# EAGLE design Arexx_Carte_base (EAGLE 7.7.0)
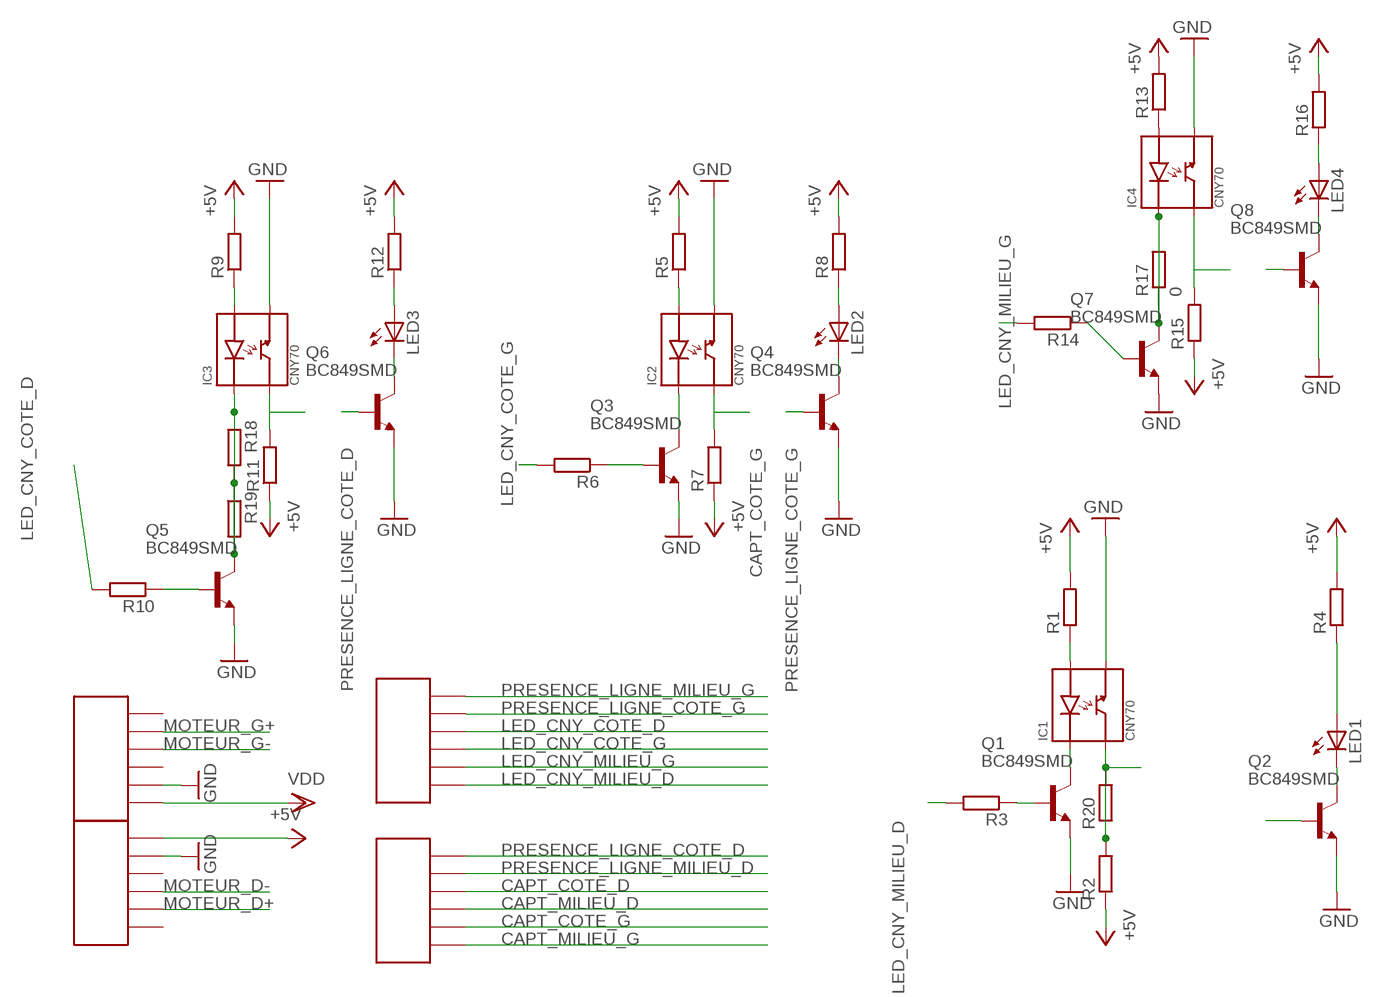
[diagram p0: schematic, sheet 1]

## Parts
IC1  CNY70  [CNY70]
IC2  CNY70  [CNY70]
IC3  CNY70  [CNY70]
IC4  CNY70  [CNY70]
LED1  LED5MM  [LED5MM]
LED2  LED5MM  [LED5MM]
LED3  LED5MM  [LED5MM]
LED4  LED5MM  [LED5MM]
Q1  BC849SMD  [SOT23-BEC]
Q2  BC849SMD  [SOT23-BEC]
Q3  BC849SMD  [SOT23-BEC]
Q4  BC849SMD  [SOT23-BEC]
Q5  BC849SMD  [SOT23-BEC]
Q6  BC849SMD  [SOT23-BEC]
Q7  BC849SMD  [SOT23-BEC]
Q8  BC849SMD  [SOT23-BEC]
R1  R-EU_R1206  [R1206]
R2  R-EU_R1206  [R1206]
R3  R-EU_R1206  [R1206]
R4  R-EU_R1206  [R1206]
R5  R-EU_R1206  [R1206]
R6  R-EU_R1206  [R1206]
R7  R-EU_R1206  [R1206]
R8  R-EU_R1206  [R1206]
R9  R-EU_R1206  [R1206]
R10  R-EU_R1206  [R1206]
R11  R-EU_R1206  [R1206]
R12  R-EU_R1206  [R1206]
R13  R-EU_R1206  [R1206]
R14  R-EU_R1206  [R1206]
R15  R-EU_R1206  [R1206]
R16  R-EU_R1206  [R1206]
R17  0  R-EU_R1206  [R1206]
R18  R-EU_R1206  [R1206]
R19  R-EU_R1206  [R1206]
R20  R-EU_R1206  [R1206]
U$1  AREXX_CONNECTEUR  [AREXX_CONNECTEUR]
U$2  AREXX_CONNECTEUR  [AREXX_CONNECTEUR]
U$3  AREXX_CONNECTEUR  [AREXX_CONNECTEUR]
U$4  AREXX_CONNECTEUR  [AREXX_CONNECTEUR]

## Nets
+5V: R1.2 R2.1 R4.2 R5.2 R7.1 R8.2 R9.2 R11.1 R12.2 R13.2 R15.1 R16.2 U$3.P$1
CAPT_COTE_D: IC3.DC R11.2 U$4.P$3
CAPT_COTE_G: IC2.DC R7.2 U$4.P$5
CAPT_MILIEU_D: IC1.DC R2.2 R20.1 R20.2 U$4.P$4
CAPT_MILIEU_G: IC4.DC R15.2 U$4.P$6
GND: IC1.DE IC2.DE IC3.DE IC4.DE Q1.E Q2.E Q3.E Q4.E Q5.E Q6.E Q7.E Q8.E U$2.P$5 U$3.P$2
LED_CNY_COTE_D: R10.2 U$1.P$3
LED_CNY_COTE_G: R6.2 U$1.P$4
LED_CNY_MILIEU_D: R3.2 U$1.P$6
LED_CNY_MILIEU_G: R14.2 U$1.P$5
MOTEUR_D+: U$3.P$5
MOTEUR_D-: U$3.P$4
MOTEUR_G+: U$2.P$2
MOTEUR_G-: U$2.P$3
N$1: Q1.B R3.1
N$2: IC1.EK Q1.C
N$3: IC1.EA R1.1
N$4: LED1.A R4.1
N$5: LED1.K(C) Q2.C
N$6: IC2.EA R5.1
N$7: IC2.EK Q3.C
N$8: Q3.B R6.1
N$9: LED2.K(C) Q4.C
N$10: LED2.A R8.1
N$11: IC3.EA R9.1
N$12: IC3.EK Q5.C R18.1 R18.2 R19.1 R19.2
N$13: Q5.B R10.1
N$14: LED3.K(C) Q6.C
N$15: LED3.A R12.1
N$16: IC4.EA R13.1
N$17: IC4.EK Q7.C R17.1 R17.2
N$18: Q7.B R14.1
N$19: LED4.K(C) Q8.C
N$21: LED4.A R16.1
PRESENCE_LIGNE_COTE_D: Q6.B U$4.P$1
PRESENCE_LIGNE_COTE_G: Q4.B U$1.P$2
PRESENCE_LIGNE_MILIEU_D: Q2.B U$4.P$2
PRESENCE_LIGNE_MILIEU_G: Q8.B U$1.P$1
VDD: U$2.P$6
Unconnected: U$2.P$1 U$2.P$4 U$3.P$3 U$3.P$6

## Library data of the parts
IC1-IC4 = CNY70:CNY70: CNY70 (Vishay) Reflexkoppler
LED1-LED4 = led:LED: LED
Q1-Q8 = transistor-npn:BC849*: NPN Transistor
R1-R20 = rcl:R-EU_: RESISTOR, European symbol
U$1-U$4 = troyesgeii:AREXX_CONNECTEUR

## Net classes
0 default: clearance 0.355 mm
2 gnd: width 0.305 mm, drill 0.559 mm, clearance 0.254 mm

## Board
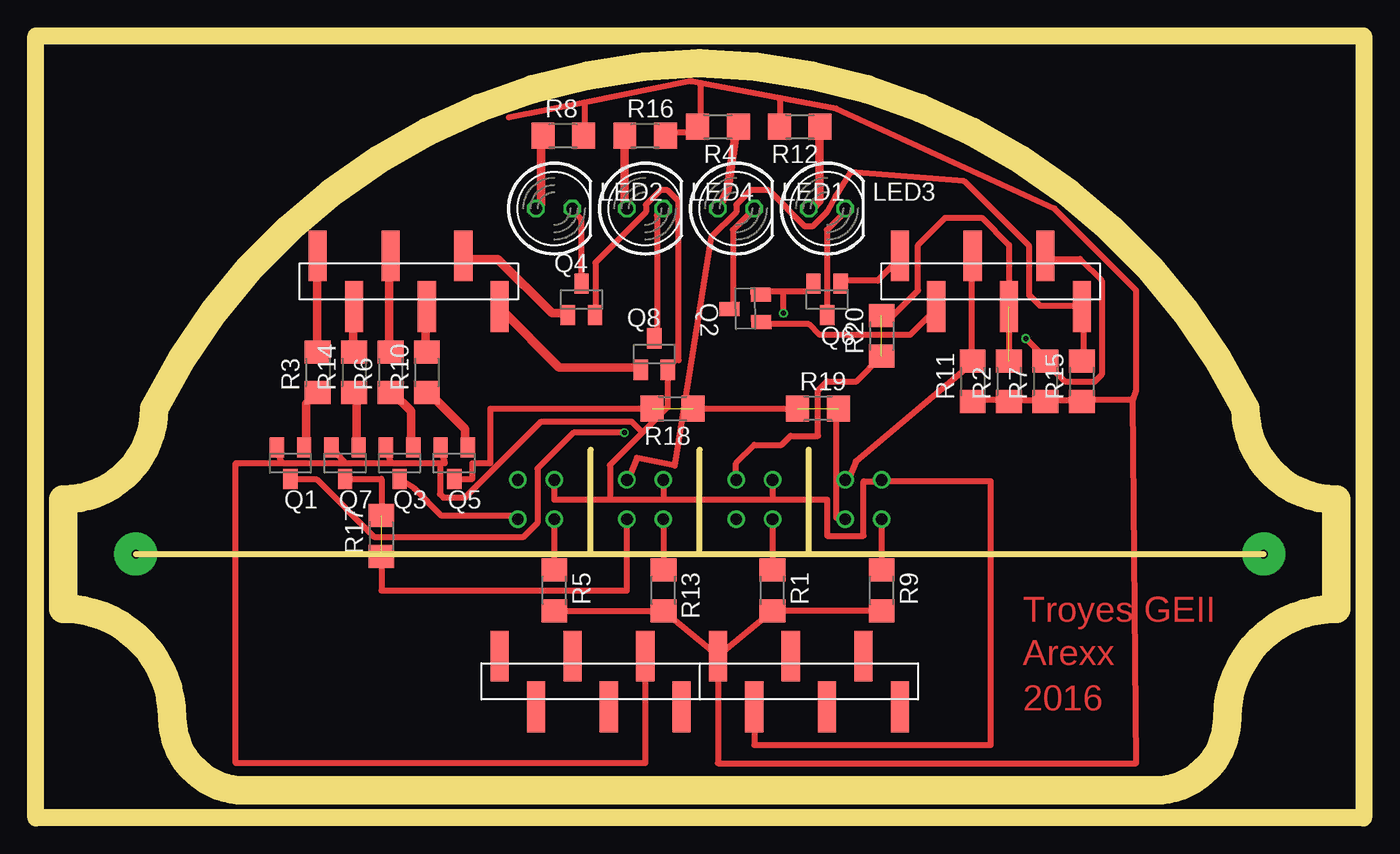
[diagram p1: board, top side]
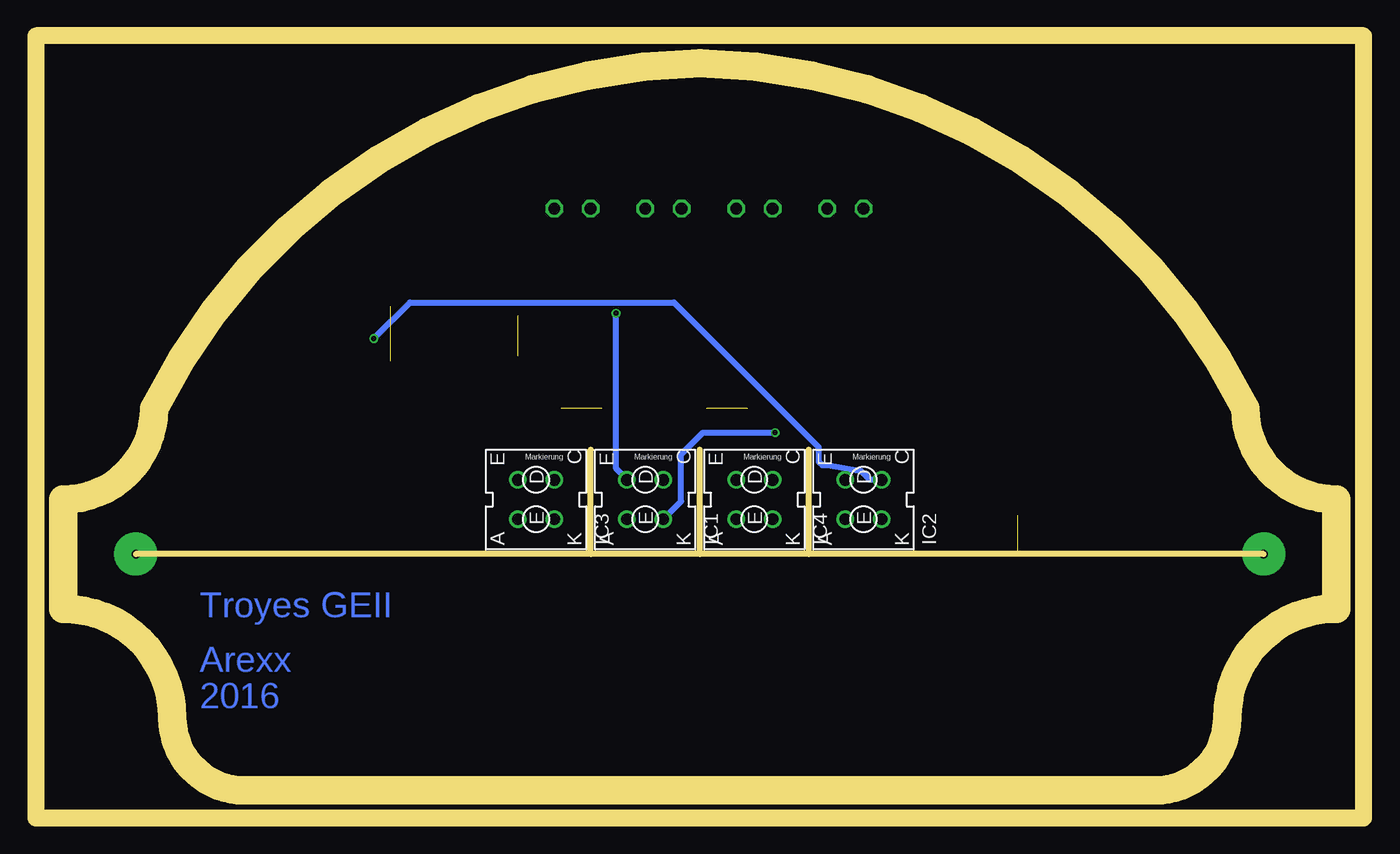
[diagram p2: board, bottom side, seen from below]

Size 92.71 x 54.61 mm. Coordinates in mm from the lower left corner, seen from the top.
Outline: 6.99,18.42 38.73,18.42
Outline: 38.73,18.42 46.35,18.42
Outline: 46.35,18.42 53.98,18.42
Outline: 53.98,18.42 85.73,18.42
Outline: 46.35,18.42 46.35,25.72
Outline: 38.73,18.42 38.73,25.72
Outline: 53.98,18.42 53.98,25.72
Outline: 0,0 0,54.61 92.71,54.61 92.71,0 0,0
Copper layers (1*16): Top 0.018mm / dielectric 1.55mm / Bottom 0.018mm
Design rules "eC_2Layer_PClass6_BaseCopperO18_eCDefault": minimum track width 0.15mm, minimum drill 0.35mm, track to track 0.15mm, track to pad 0.15mm, pad to pad 0.15mm, via to via 0.15mm, smd to smd 0mil, copper to edge 0.25mm, drill to drill 0.35mm, minimum pad ring 0.175mm, minimum via ring 0.125mm, stop-mask expansion 0mil, vias tented up to drill 0.45mm, thermal gap 0.2mm
Milling: 11 lines

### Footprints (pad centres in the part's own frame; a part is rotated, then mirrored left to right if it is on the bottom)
CNY70 = drill 0.813: DC 1.37,-1.27; DE 1.37,1.27; EA -1.37,1.27; EK -1.37,-1.27
LED5MM = drill 0.813 octagon: A -1.27,0; K 1.27,0
SOT23-BEC = smd 1 x 1.4: B -0.95,-1.1; C 0,1.1; E 0.95,-1.1
R1206 = smd 1.6 x 1.803: 1 -1.422,0; 2 1.422,0
AREXX_CONNECTEUR = smd 1.27 x 3.54: P$1 -6.35,1.77; P$2 -3.81,-1.77; P$3 -1.27,1.77; P$4 1.27,-1.77; P$5 3.81,1.77; P$6 6.35,-1.77

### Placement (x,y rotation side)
IC1  50.16,22.23 90 bottom
IC2  34.92,22.23 90 bottom
IC3  57.78,22.23 90 bottom
IC4  42.55,22.23 90 bottom
LED1  48.89,42.55 0 top
LED2  36.2,42.55 0 top
LED3  55.24,42.55 0 top
LED4  42.55,42.55 0 top
Q1  17.78,24.77 180 top
Q2  49.53,35.56 91 top
Q3  25.4,24.77 180 top
Q4  38.1,36.2 0 top
Q5  29.21,24.77 180 top
Q6  55.24,36.2 180 top
Q7  21.59,24.77 180 top
Q8  43.18,32.38 0 top
R1  51.43,15.88 270 top
R2  67.95,30.48 90 top
R3  19.69,31.12 90 top
R4  47.62,48.26 180 top
R5  36.2,15.88 270 top
R6  24.77,31.12 90 top
R7  70.48,30.48 90 top
R8  36.83,47.62 0 top
R9  59.05,15.88 270 top
R10  27.3,31.12 90 top
R11  65.41,30.48 90 top
R12  53.34,48.26 180 top
R13  43.81,15.88 270 top
R14  22.23,31.12 90 top
R15  73.03,30.48 90 top
R16  42.55,47.62 0 top
R17  24.13,19.69 90 top
R18  44.45,28.58 180 top
R19  54.61,28.58 0 top
R20  59.05,33.66 90 top
U$1  26.04,37.47 180 top
U$2  38.73,9.53 0 top
U$3  53.98,9.53 0 top
U$4  66.67,37.47 0 top

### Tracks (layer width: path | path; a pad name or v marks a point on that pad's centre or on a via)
+5V
  Top 0.15: 65.58,29.18 R11.1 | 67.85,29.18 R2.1 68.11,29.18 | 70.38,29.18 R7.1 70.63,29.18 | 72.9,29.18 R15.1 73.16,29.18 | 45.88,47.86 46.14,48.11 R4.2 46.39,48.37 | 44.12,47.86 R16.2 | 38.31,47.86 R8.2 | 38.31,49.88 38.3,49.95 | 51.95,50.13 51.97,50.26 | 46.39,51.14 46.42,51.3 | 76.44,29.18 76.58,29.12
  Top 0.406: U$3.P$1 47.62,3.81 76.84,3.81 76.58,29.12 76.84,29.85 76.84,36.83 71.12,42.55 55.88,49.53 51.97,50.26 46.42,51.3 45.72,51.44 38.3,49.95 33.02,48.9 | R5.2 R13.2 U$3.P$1 | U$3.P$1 R1.2 R9.2 | 67.85,29.18 65.58,29.18 | 68.11,29.18 70.38,29.18 | 70.63,29.18 72.9,29.18 | 45.88,47.86 44.12,47.86 | 38.31,49.88 38.31,47.86 | 51.95,50.13 51.95,48.37 R12.2 | 46.39,51.14 46.39,48.37 | 76.44,29.18 73.16,29.18
CAPT_COTE_D
  Top 0.15: 65.33,31.95 R11.2 65.33,31.7 | 65.33,39.02 U$4.P$3
  Top 0.406: 65.33,39.02 65.33,31.95 | 65.33,31.7 57.25,24.89 56.74,23.62 IC3.DC
CAPT_COTE_G  (via drill 0.35)
  Top 0.15: 70.63,31.7 R7.2 70.63,31.95 | 70.63,39.02 U$4.P$5
  Top 0.406: 70.63,31.7 71.89,30.44 73.91,30.44 74.42,30.94 74.42,37.51 72.9,39.02 70.63,39.02 | 70.63,31.95 v69.12,33.47
  Bottom 0.15: 33.77,23.62 IC2.DC
  Bottom 0.406: 33.77,23.62 34.52,23.62 35.15,24.25 35.27,24.25 37.43,24.63 37.8,24.63 38.06,24.88 38.06,25.89 48.16,35.99 66.59,35.99 v69.12,33.47
CAPT_MILIEU_D  (2 unrouted)
  Top 0.406: IC1.DC 48.89,24.77 50.16,26.04 52.07,26.04 52.7,26.67 54.61,26.67 54.61,29.85 55.24,30.48 57.3,30.48 R20.1 | R20.2 59.84,35.08 61.59,36.83 61.59,40.01 63.5,41.91 66.04,41.91 67.95,40.01 R2.2
CAPT_MILIEU_G
  Top 0.15: 73.16,31.95 R15.2 | 73.16,35.49 U$4.P$6 72.9,35.74
  Top 0.406: 73.16,35.49 73.16,31.95 | 72.9,35.74 70.12,35.74 69.37,36.5 69.37,39.91 64.82,44.45 56.87,45.09 55.86,43.45 55.23,42.3 54.22,41.3 53.71,41.3 51.19,43.82 49.92,43.82 48.91,42.81 48.91,42.3 47.15,40.54 44.61,24.59 41.98,25.14 41.34,23.62 IC4.DC
GND  (via drill 0.35)
  Top 0.15: 53.71,36.75 54.22,37.26 Q6.E | 50.68,36.75 Q2.E | 44.88,31.95 44.37,31.45 Q8.E 44.12,31.2 | 39.07,35.23 Q4.E
  Top 0.406: U$2.P$5 42.55,3.81 13.97,3.81 13.97,24.77 17.14,24.77 | 17.14,24.77 21.59,24.77 | 21.59,24.77 24.77,24.77 | 24.77,24.77 28.21,24.77 | 28.21,24.77 28.58,24.77 Q5.E | Q1.E 17.14,24.77 | Q7.E 21.59,24.77 | Q3.E 24.77,24.77 | IC2.DE 36.2,22.23 40.08,22.23 | 40.08,22.23 43.81,22.23 | 43.81,22.23 51.43,22.23 | 51.43,22.23 55.24,22.23 55.24,19.69 57.78,19.69 57.78,23.5 59.05,23.5 | IC4.DE 43.81,22.23 | IC1.DE 51.43,22.23 | U$3.P$2 50.16,5.08 66.67,5.08 66.67,23.5 59.05,23.5 | 53.71,36.75 52.2,36.75 | 52.2,36.75 50.68,36.75 | v52.2,35.23 52.2,36.75 | 39.07,35.23 39.07,38.77 42.6,42.3 42.6,42.81 43.61,43.82 44.12,43.82 44.88,43.06 44.88,31.95 | 40.08,22.23 40.08,24.63 42.35,26.9 | 42.35,26.9 44.12,28.67 44.12,31.2 | 42.35,26.9 41.59,27.66 35.28,27.66 29.98,22.36 28.46,22.36 28.21,22.61 28.21,24.77 | 59.05,23.5 IC3.DE
  Bottom 0.15: 51.44,23.62 IC1.DE
  Bottom 0.406: v52.2,35.23 52.2,24.38 51.44,23.62
LED_CNY_COTE_D
  Top 0.15: 27.2,32.71 R10.2 | 27.2,35.49 U$1.P$3
  Top 0.61: 27.2,35.49 27.2,32.71
LED_CNY_COTE_G
  Top 0.15: 24.68,32.71 R6.2 | 24.68,39.02 U$1.P$4
  Top 0.61: 24.68,39.02 24.68,32.71
LED_CNY_MILIEU_D
  Top 0.15: 19.62,32.71 R3.2 | 19.62,39.02 U$1.P$6
  Top 0.61: 19.62,39.02 19.62,32.71
LED_CNY_MILIEU_G
  Top 0.15: 22.15,32.71 R14.2 | 22.15,35.49 U$1.P$5
  Top 0.61: 22.15,35.49 22.15,32.71
N$1
  Top 0.15: 18.87,28.92 19.62,29.68 R3.1 | 18.87,25.89 Q1.B
  Top 0.61: 18.87,28.92 18.87,25.89
N$2  (via drill 0.35)
  Top 0.15: 17.86,23.62 Q1.C
  Top 0.406: 17.86,23.62 19.62,23.62 23.66,19.58 34.02,19.58 35.03,20.59 35.03,24.38 37.55,26.9 v41.09,26.9
  Bottom 0.406: v41.09,26.9 46.14,26.9 47.65,25.39 47.65,22.11 48.66,21.1 IC1.EK
N$3
  Top 0.406: IC1.EA R1.1
N$4
  Top 0.15: 47.65,42.56 LED1.A
  Top 0.406: 48.91,48.11 R4.1
  Top 0.61: 48.91,48.11 48.28,43.82 47.65,42.56
N$5
  Top 0.15: 48.66,35.74 Q2.C
  Top 0.406: 48.66,35.74 48.66,41.04 LED1.K
N$6
  Top 0.406: IC2.EA R5.1
N$7
  Top 0.15: 25.43,23.62 Q3.C
  Top 0.406: 25.43,23.62 26.44,22.98 28.33,21.1 33.51,21.1 IC2.EK
N$8
  Top 0.15: 26.19,25.89 Q3.B | 24.93,29.68 R6.1
  Top 0.61: 26.19,25.89 26.19,28.42 24.93,29.68
N$9
  Top 0.15: 38.06,37.51 Q4.C | 37.55,42.3 LED2.K
  Top 0.406: 38.06,37.51 38.06,41.8 37.55,42.3
N$10
  Top 0.15: 35.03,42.56 35.28,42.81 | 35.28,47.61 R8.1
  Top 0.406: 35.03,42.56 LED2.A
  Top 0.61: 35.28,42.81 35.28,47.61
N$11
  Top 0.406: IC3.EA R9.1
N$12  (2 unrouted)
  Top 0.406: Q5.C 30.48,23.67 30.48,24.77 31.75,24.77 31.75,28.58 R18.2 | R18.1 R19.1 | R19.2 55.88,28.58 55.88,20.96 56.52,20.96 IC3.EK
N$13
  Top 0.15: 29.98,25.89 Q5.B | 27.45,29.68 R10.1
  Top 0.61: 29.98,25.89 29.98,27.16 27.45,29.68
N$14
  Top 0.15: 55.23,35.23 Q6.C
  Top 0.406: 55.23,35.23 55.23,41.04 56.49,42.3 LED3.K
N$15
  Top 0.406: 54.72,48.11 R12.1
  Top 0.61: 54.72,48.11 54.72,43.06 54.22,42.56 LED3.A
N$16
  Top 0.406: IC4.EA R13.1
N$17  (1 unrouted)
  Top 0.406: Q7.C 24.13,23.67 R17.2 | R17.1 24.13,15.88 41.27,15.88 IC4.EK
N$18
  Top 0.15: 22.4,25.89 Q7.B | 22.4,29.68 R14.1
  Top 0.61: 22.4,29.68 22.4,25.89
N$19
  Top 0.15: 43.36,42.05 43.61,42.3 LED4.K | 43.36,33.72 Q8.C
  Top 0.406: 43.36,42.05 43.36,33.72
N$20  (via drill 0.6 pad 3)
  other vias: 6.99,18.42
N$21
  Top 0.15: 41.09,47.61 R16.1 | 41.09,42.56 LED4.A
  Top 0.61: 41.09,42.56 41.09,47.61
N$24  (via drill 0.6 pad 3)
  other vias: 85.73,18.42
PRESENCE_LIGNE_COTE_D
  Top 0.15: 56.24,37.51 Q6.B | 60.28,39.02 U$4.P$1
  Top 0.406: 56.24,37.51 58.76,37.51 60.28,39.02
PRESENCE_LIGNE_COTE_G
  Top 0.15: 37.05,35.23 Q4.B | 29.98,39.02 U$1.P$2
  Top 0.61: 37.05,35.23 36.04,35.23 32.25,39.02 29.98,39.02
PRESENCE_LIGNE_MILIEU_D
  Top 0.15: 50.68,34.48 Q2.B | 62.8,35.49 U$4.P$2
  Top 0.406: 50.68,34.48 53.96,34.48 54.72,33.72 61.03,33.72 62.8,35.49
PRESENCE_LIGNE_MILIEU_G
  Top 0.15: 42.1,31.45 Q8.B | 32.5,35.49 U$1.P$1
  Top 0.61: 42.1,31.45 36.54,31.45 32.5,35.49

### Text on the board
Top: Troyes GEII | Arexx | 2016
Bottom: Troyes GEII | Arexx | 2016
